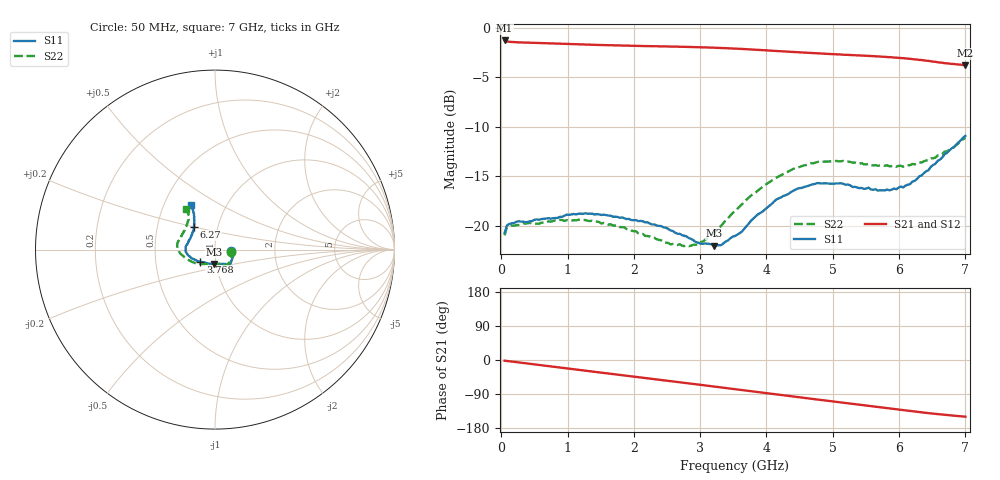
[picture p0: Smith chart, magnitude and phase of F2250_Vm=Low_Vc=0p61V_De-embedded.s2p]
! Integrated Device Technology
! Corporate Headquarters
! 6024 Silver Creek Valley Road
! San Jose, CA 95138  USA
! Phone:  1-408-284-8200
! Toll Free:  1-800-223-1366
! Webpage:  http://www.idt.com/
! Timing and RF Division
! 515 Groton Road, Suite 102
! Westford, MA 01886-6024
! Device:  F2250
! Description: Voltage Variable RF Attenuator
! Frequency:  50.0 -  6000.00 MHz
! Package:  3x3 mm Thin QFN Plastic Package: 16 pin
! Ports:  2 RF, 3 DC
!  Pin  1  = GND
!  Pin  2  = NC
!  Pin  3  = RF1  = Port 1
!  Pin  4  = NC
!  Pin  5  = GND
!  Pin  6  = GND
!  Pin  7  = GND
!  Pin  8  = GND
!  Pin  9  = NC
!  Pin 10  = RF2  = Port 2
!  Pin 11  = NC
!  Pin 12  = GND
!  Pin 13  = GND
!  Pin 14  = VCNTRL
!  Pin 15  = VDD
!  Pin 16  = VMODE
! Vcntrl:  0.610 Volts
! Vmode:  +0.000 Volts
! Vdd:  +3.30  Volts
! Current:  1.139 mA
! Data:  The device was measured on a the F2250 evaluation board which has
!  individual transmission lines to the RF pins.  Data was collected
!  using a calibrated network analyzer.  The evaluation board was
!  de-embedded using a TRL calibration technique.
!  The reference plane is the edge of the package pin.
! Misc:  SN 10
!  Action Tracker AT0258
! Date Measured:  2014-11-26
! Date:  2015-10-15  MJV
! Note:
!  Integrated Device Technology supplies this data as a sample of measured
!  data at the package pin for this product.  Your particular data for this
!  product may vary.
!  Data was taken at 25 degrees C.
!  Integrated Device Technology reserves the right to change this data at anytime.
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# GHz S dB R 50
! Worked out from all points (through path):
!   201 points, 50 MHz to 7 GHz, reference 50 ohm
!   highest |S21| = -1.29 dB at 50 MHz (marker M1); lowest = -3.8 dB at 7 GHz (marker M2)
!   group delay of S21, straight-line fit = 60.1 ps
!   lowest |S11| = -22.0 dB at 3.212 GHz (marker M3), VSWR 1.17, Z = 48.9 - j7.81 ohm
!   |S11| at or under -10 dB: start of sweep to end of sweep
!   |S22| runs from -22.0 to -11.1 dB; largest |S21 - S12| = 0.00054
!   S11 on the Smith chart (normalised r, x): 50 MHz: 1.20, -0.02; 3.768 GHz: 0.84, -0.12; 6.27 GHz: 0.77, +0.20; 7 GHz: 0.68, +0.37
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0.05  -20.70 -5.8  -1.29 -1.8  -1.29 -1.8  -20.94 -7.0
0.08475  -19.94 -6.0  -1.39 -2.5  -1.39 -2.5  -20.15 -6.8
0.328  -19.55 -13.5  -1.50 -7.8  -1.50 -7.8  -19.73 -15.3
0.77975  -19.22 -30.4  -1.59 -17.7  -1.59 -17.7  -19.50 -35.1
1.2315  -18.78 -43.4  -1.70 -27.4  -1.70 -27.4  -19.42 -52.0
1.75275  -19.08 -50.3  -1.80 -38.5  -1.79 -38.5  -19.93 -62.2
2.37825  -19.99 -53.4  -1.88 -51.8  -1.88 -51.8  -21.40 -71.5
2.83  -21.22 -66.3  -1.95 -61.7  -1.95 -61.7  -22.03 -92.4
3.0385  -21.80 -80.0  -1.98 -66.3  -1.98 -66.3  -21.58 -107.2
3.21225  -21.99 -93.7  -2.02 -70.2  -2.02 -70.2  -20.66 -119.8
3.3165  -21.93 -104.2  -2.05 -72.5  -2.05 -72.5  -19.98 -126.6
3.525  -21.01 -122.2  -2.11 -77.2  -2.11 -77.2  -18.50 -138.7
3.76825  -19.45 -140.5  -2.20 -82.6  -2.20 -82.6  -16.92 -150.2
4.1505  -17.32 -158.3  -2.36 -91.0  -2.35 -91.0  -15.12 -166.0
4.46325  -16.23 -168.5  -2.48 -97.7  -2.48 -97.8  -14.11 -174.9
4.7065  -15.79 -175.4  -2.57 -103.0  -2.57 -103.0  -13.67 179.5
5.15825  -15.75 173.6  -2.73 -112.7  -2.73 -112.7  -13.44 169.6
5.85325  -16.40 149.6  -2.98 -127.6  -2.98 -127.6  -13.98 153.6
6.06175  -16.11 141.1  -3.08 -132.1  -3.08 -132.1  -14.02 147.6
6.27025  -15.25 132.7  -3.22 -136.7  -3.22 -136.7  -13.71 141.0
6.61775  -13.30 122.0  -3.52 -143.4  -3.52 -143.4  -12.86 129.3
7  -10.92 118.1  -3.79 -149.5  -3.79 -149.6  -11.11 125.0
